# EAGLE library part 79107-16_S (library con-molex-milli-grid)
RECEPTACAL
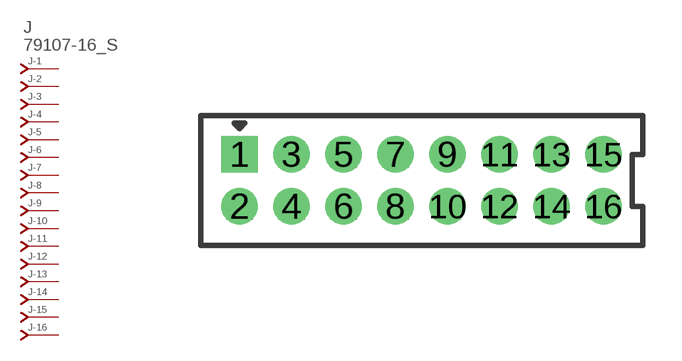
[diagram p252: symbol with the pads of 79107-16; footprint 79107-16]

Designator prefix J; gates -1=J-NV -2=J-N -3=J-N -4=J-N -5=J-N -6=J-N -7=J-N -8=J-N -9=J-N -10=J-N -11=J-N -12=J-N -13=J-N -14=J-N -15=J-N -16=J-N

## 79107-16_S  [79107-16]
1  -1:J  pas
2  -2:J  pas
3  -3:J  pas
4  -4:J  pas
5  -5:J  pas
6  -6:J  pas
7  -7:J  pas
8  -8:J  pas
9  -9:J  pas
10  -10:J  pas
11  -11:J  pas
12  -12:J  pas
13  -13:J  pas
14  -14:J  pas
15  -15:J  pas
16  -16:J  pas

## Footprint 79107-16 (pad centres in mm)
RECEPTACAL Dual Row, Vertical, Through-Hole
drill 0.914 square: 1 -7,1
drill 0.914: 2 -7,-1; 3 -5,1; 4 -5,-1; 5 -3,1; 6 -3,-1; 7 -1,1; 8 -1,-1; 9 1,1; 10 1,-1; 11 3,1; 12 3,-1; 13 5,1; 14 5,-1; 15 7,1; 16 7,-1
